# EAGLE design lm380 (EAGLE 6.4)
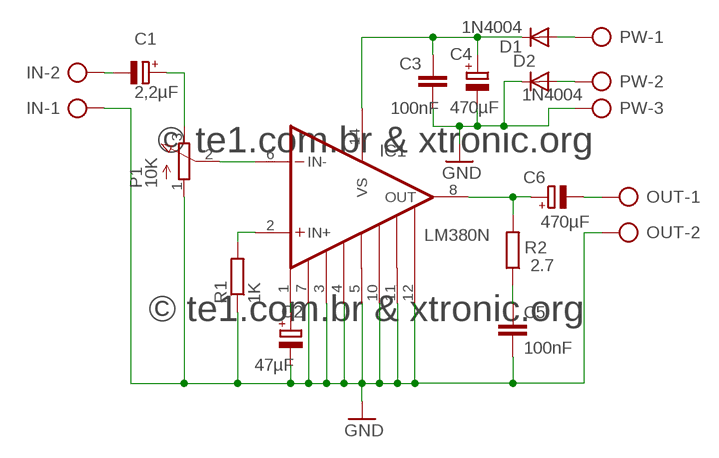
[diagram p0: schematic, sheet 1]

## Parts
C1  2,2µF  CPOL-EUE2-4  [E2-4]
C2  47µF  CPOL-EUE2-4  [E2-4]
C3  100nF  C-EU050-025X075  [C050-025X075]
C4  470µF  CPOL-EUE2.5-7  [E2,5-7]
C5  100nF  C-EU050-025X075  [C050-025X075]
C6  470µF  CPOL-EUE2.5-7  [E2,5-7]
D1  1N4004  [DO41-10]
D2  1N4004  [DO41-10]
IC1  LM380N  [DIL14]
IN  AK500/2-H  [AK500/2-H]
OUT  AK500/2-H  [AK500/2-H]
P1  10K  3RP/1610N  [3RP/1610N]
PW  AK500/3-H  [AK500/3-H]
R1  1K  R-EU_0207/10  [0207/10]
R2  2.7  R-EU_0207/10  [0207/10]

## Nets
GND: C2.- C3.2 C4.- C5.2 D2.C IC1.3 IC1.4 IC1.5 IC1.7 IC1.10 IC1.11 IC1.12 IN.1 OUT.2 P1.1(A) PW.3 R1.1
N$1: IC1.6(IN-) P1.2(S)
N$2: IC1.2(IN+) R1.2
N$3: C6.+ IC1.8(OUT) R2.2
N$4: C5.1 R2.1
N$5: D1.A PW.1
N$6: C2.+ IC1.1(BYPASS)
N$7: C1.+ P1.3(E)
N$8: C1.- IN.2
N$9: C6.- OUT.1
N$11: C3.1 C4.+ D1.C IC1.14(VS)
N$13: D2.A PW.2

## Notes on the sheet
- © te1.com.br & xtronic.org
- © te1.com.br & xtronic.org

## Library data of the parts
C1 C2 C4 C6 = rcl:CPOL-EU: POLARIZED CAPACITOR, European symbol
C3 C5 = rcl:C-EU: CAPACITOR, European symbol
D1 D2 = diode:1N4004: DIODE
IC1 = lm380:LM380N
IN OUT = con-ptr500:AK500/2-H: CONNECTOR; OC_FARNELL: unknown; OC_NEWARK: unknown
P1 = pot:3RP/1610N: 16mm Potentiometer one level Source: http://www.alphapotentiometers.net/html/16mm_pot_2.html
PW = con-ptr500:AK500/3-H: CONNECTOR Aug. 2004 / PTR Meßtechnik: Die Bezeichnung der Serie AK505 wurde geändert. Es handelt sich hierbei um AK500 in horizontaler Ausführung.; OC_FARNELL: unknown; OC_NEWARK: unknown
R1 R2 = rcl:R-EU_: RESISTOR, European symbol

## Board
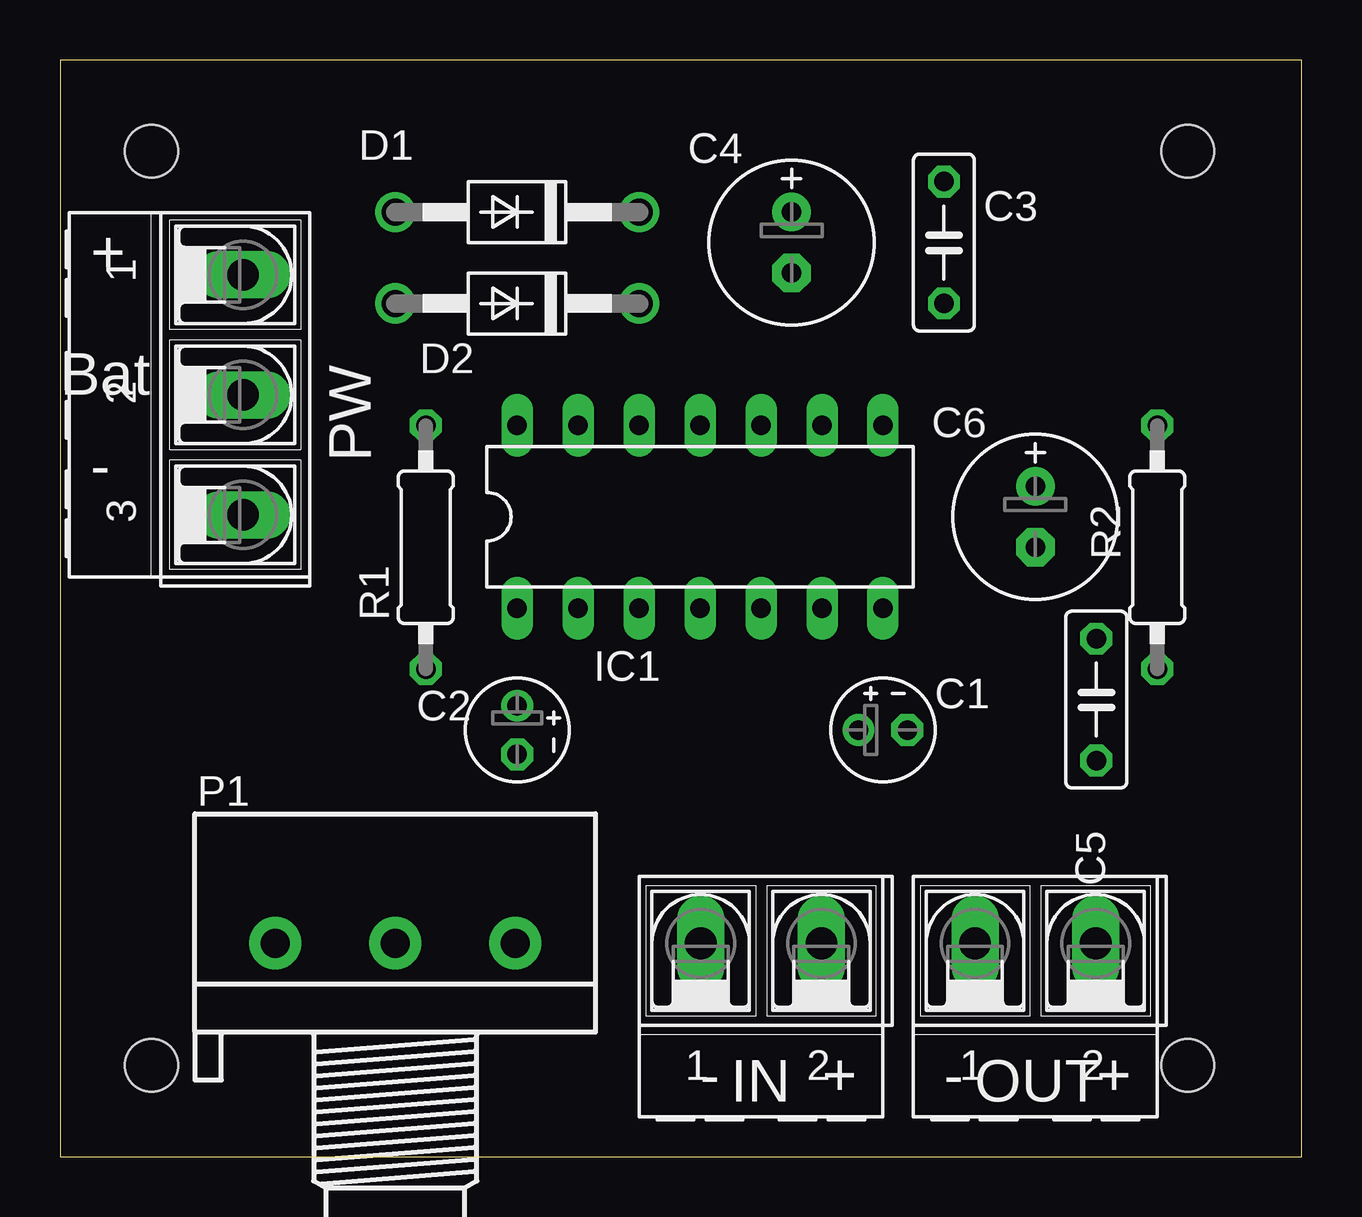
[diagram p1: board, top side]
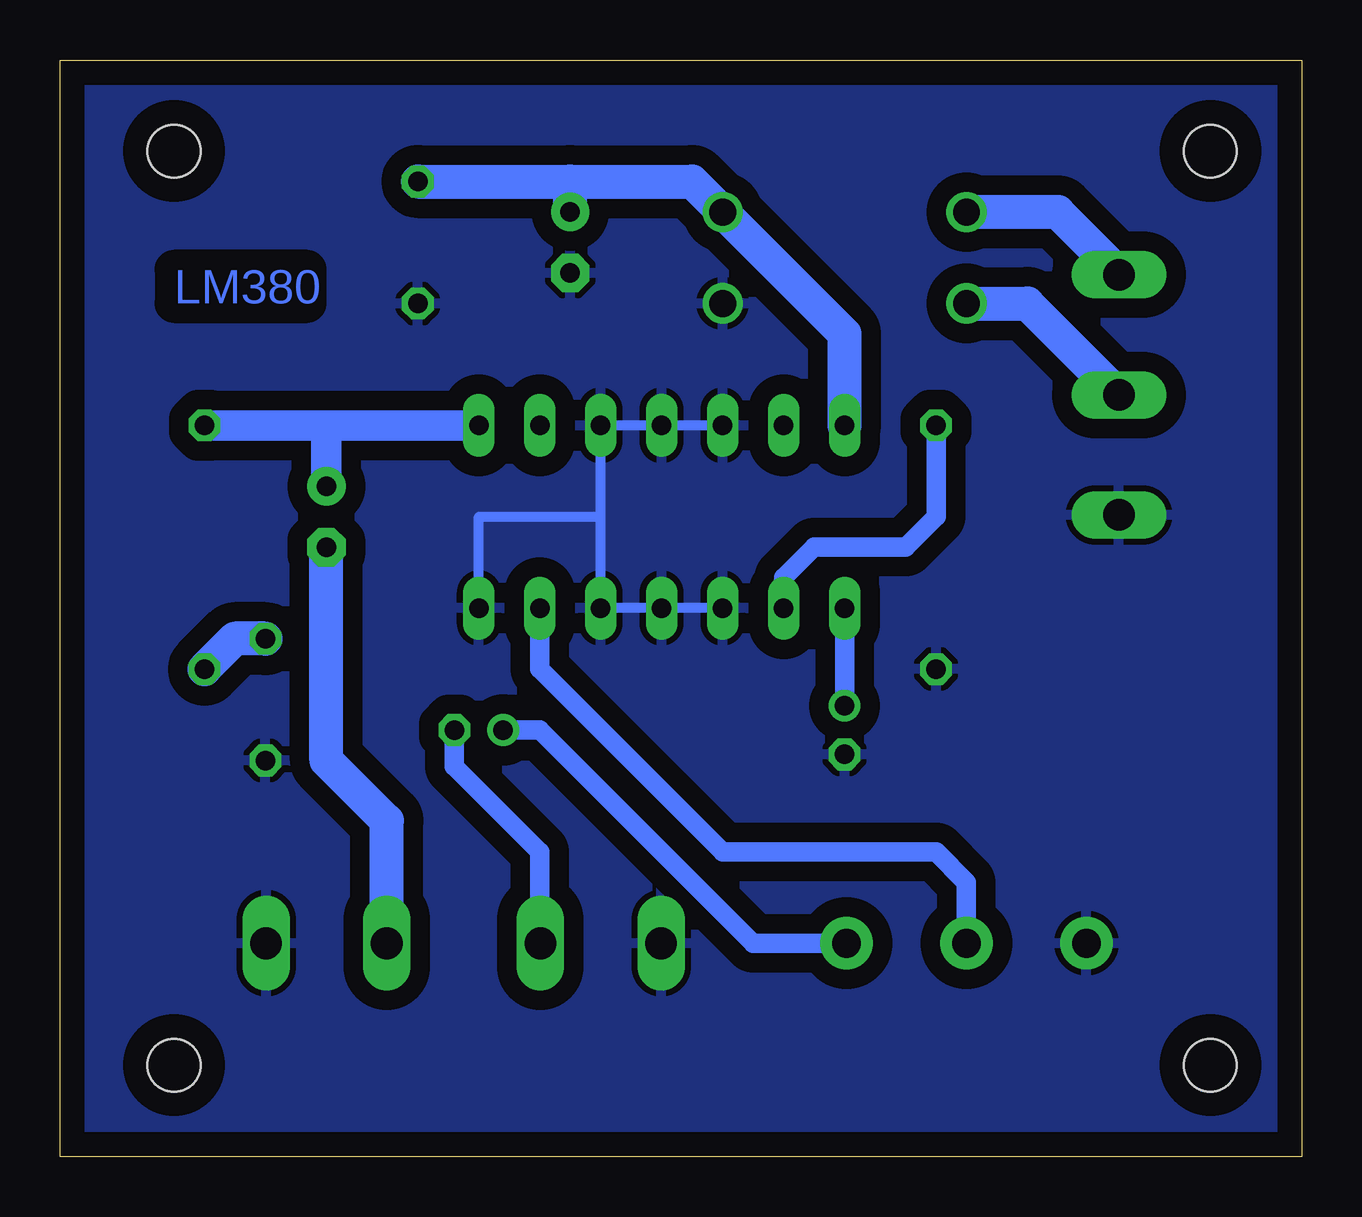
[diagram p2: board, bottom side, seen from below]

Size 51.74 x 45.71 mm. Coordinates in mm from the lower left corner, seen from the top.
Outline: 0,0 51.74,0 51.74,45.71 0,45.71 0,0
Copper layers (1*16): Top 0.035mm / dielectric 1.5mm / Bottom 0.035mm
Design rules "default": minimum track width 10mil, minimum drill 24mil, track to track 8mil, track to pad 8mil, pad to pad 8mil, via to via 8mil, smd to smd 8mil, copper to edge 40mil, drill to drill 8mil, minimum pad ring 10mil, minimum via ring 8mil, stop-mask expansion 4mil, vias tented up to drill 0mil, thermal gap 10mil
Holes 2.2 mm at 3.81,41.91 46.99,41.91 46.99,3.81 3.81,3.81

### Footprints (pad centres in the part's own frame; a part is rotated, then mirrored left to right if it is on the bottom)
E2-4 = drill 0.813 pad 1.27: + -1.016,0 | drill 0.813 pad 1.27 octagon: - 1.016,0
C050-025X075 = drill 0.813 octagon: 1 -2.54,0; 2 2.54,0
E2,5-7 = drill 0.813 pad 1.6: + -1.27,0 | drill 0.813 pad 1.6 octagon: - 1.27,0
DO41-10 = drill 1.118: A 5.08,0; C -5.08,0
DIL14 = drill 0.813 long: 1 -7.62,-3.81; 2 -5.08,-3.81; 3 -2.54,-3.81; 4 0,-3.81; 5 2.54,-3.81; 6 5.08,-3.81; 7 7.62,-3.81; 8 7.62,3.81; 9 5.08,3.81; 10 2.54,3.81; 11 0,3.81; 12 -2.54,3.81; 13 -5.08,3.81; 14 -7.62,3.81
AK500/2-H = drill 1.321 long: 1 -2.515,0; 2 2.515,0
3RP/1610N = drill 1.2 pad 2.184: 1 -5,0; 2 0,0; 3 5,0
AK500/3-H = drill 1.321 long: 1 -5.004,0; 2 0,0; 3 5.004,0
0207/10 = drill 0.813 octagon: 1 -5.08,0; 2 5.08,0

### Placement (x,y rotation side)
C1  34.29,17.78 0 top
C2  19.05,17.78 270 top
C3  36.83,38.1 270 top
C4  30.48,38.1 270 top
C5  43.18,19.05 270 top
C6  40.64,26.67 270 top
D1  19.05,39.37 180 top
D2  19.05,35.56 180 top
IC1  26.67,26.67 0 top
IN  29.21,8.89 0 top
OUT  40.64,8.89 0 top
P1  13.97,8.89 0 top
PW  7.62,31.75 270 top
R1  15.24,25.4 90 top
R2  45.72,25.4 90 top

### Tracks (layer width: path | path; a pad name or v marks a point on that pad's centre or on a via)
GND
  Bottom 0.406: IC1.12 IC1.11 IC1.10 29.21,26.67 | 29.21,26.67 IC1.5 IC1.4 IC1.3 | IC1.7 34.29,26.67 29.21,26.67
  pour Bottom (isolate 0.813): 0,45.72 0,0 53.34,0 53.34,45.72
N$1
  Bottom 0.813: P1.2 13.97,11.43 15.24,12.7 24.13,12.7 31.75,20.32 IC1.6
N$2
  Bottom 0.813: IC1.2 21.59,24.13 20.32,25.4 16.51,25.4 15.24,26.67 R1.2
N$3
  Bottom 1.27: IC1.8 40.64,30.48 | 40.64,30.48 R2.2 | C6.+ 40.64,30.48
N$4
  Bottom 1.422: C5.1 44.45,21.59 R2.1
N$5
  Bottom 1.422: D1.A 10.16,39.37 7.62,36.83 PW.1
N$6
  Bottom 0.813: IC1.1 C2.+
N$7
  Bottom 0.813: P1.3 22.86,8.89 31.75,17.78 C1.+
N$8
  Bottom 0.813: C1.- 35.31,16.26 31.75,12.7 31.75,8.91 IN.2
N$9
  Bottom 1.422: OUT.1 38.12,13.99 40.64,16.51 C6.-
N$11
  Bottom 1.422: IC1.14 19.05,34.29 D1.C 25.4,40.64 30.48,40.64 | C3.1 30.48,40.64 | C4.+ 30.48,40.64
N$13
  Bottom 1.422: D2.A 11.43,35.56 PW.2

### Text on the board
Bottom: LM380
tNames: + | Bat | - | - | + | - | +
Holes: LM380 | © te1.com.br | © xtronic.org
